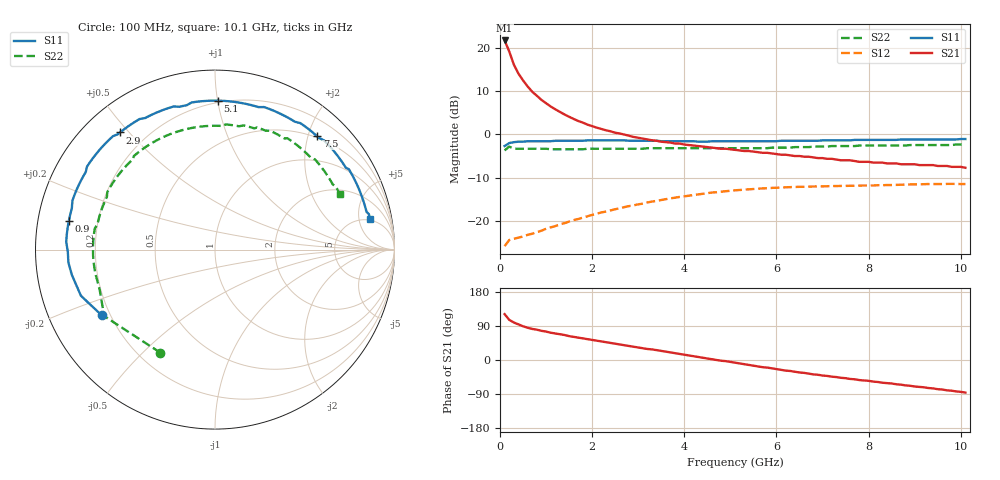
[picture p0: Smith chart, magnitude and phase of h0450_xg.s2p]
!HBFP-0450
!S and NOISE PARAMETERS at Vce=0.5V  Ic=35mA.  LAST UPDATED  09-04-98
# GHZ S MA R  50
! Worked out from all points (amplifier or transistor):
!   101 points, 100 MHz to 10.1 GHz, reference 50 ohm
!   highest |S21| = 21.6 dB at 100 MHz (marker M1)
!   |S21| within 3 dB of that: start of sweep to 215.6 MHz
!   unconditionally stable (mu >= 1): 1.433 GHz to end of sweep
!   at 1.7 GHz: K = 1.06, MAG = 9.9 dB, |S12| = -19.6 dB
!   at 5.1 GHz: K = 1.15, MAG = 2.3 dB, |S12| = -13.0 dB
!   at 10.1 GHz: K = 1.12, MAG = -0.3 dB, |S12| = -11.5 dB
!   lowest NFmin = 1.72 dB at 1.8 GHz
!   S11 on the Smith chart (normalised r, x): 100 MHz: 0.17, -0.26; 900 MHz: 0.09, +0.10; 2.9 GHz: 0.11, +0.47; 5.1 GHz: 0.19, +1.00; 7.5 GHz: 0.47, +2.16; 10.1 GHz: 4.83, +7.19
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0.1  0.73 -150.0  12.09 121.0  0.051 30.0  0.65 -118.0
0.2  0.79 -161.0  9.04 106.0  0.06 22.0  0.72 -149.0
0.3  0.81 -170.0  6.37 99.0  0.062 20.0  0.68 -161.0
0.4  0.82 -175.0  5.01 94.0  0.064 20.0  0.68 -169.0
0.5  0.82 -179.0  4.18 89.0  0.066 21.0  0.68 -174.0
0.6  0.83 177.0  3.56 85.0  0.069 21.0  0.68 -177.0
0.7  0.83 174.0  3.09 82.0  0.071 23.0  0.68 179.0
0.9  0.83 169.0  2.49 77.0  0.077 25.0  0.68 173.0
1.1  0.83 164.0  2.09 72.0  0.084 27.0  0.67 168.0
1.3  0.84 159.0  1.81 68.0  0.091 28.0  0.67 163.0
1.5  0.84 155.0  1.59 63.0  0.098 28.0  0.67 159.0
1.8  0.84 149.0  1.36 57.0  0.109 28.0  0.67 154.0
2.3  0.85 139.0  1.11 47.0  0.128 26.0  0.68 145.0
2.9  0.84 129.0  0.93 35.0  0.151 21.0  0.68 136.0
3.5  0.83 118.0  0.82 24.0  0.174 14.0  0.69 126.0
4.4  0.82 102.0  0.72 6.0  0.205 2.0  0.69 111.0
5.1  0.83 89.0  0.66 -7.0  0.225 -8.0  0.69 99.0
5.7  0.83 78.0  0.61 -19.0  0.237 -17.0  0.69 88.0
6.8  0.84 59.0  0.54 -38.0  0.249 -33.0  0.72 71.0
7.5  0.85 48.0  0.5 -48.0  0.253 -43.0  0.73 61.0
8.5  0.86 34.0  0.46 -62.0  0.259 -55.0  0.74 48.0
10.1  0.88 11.0  0.41 -86.0  0.266 -78.0  0.76 24.0
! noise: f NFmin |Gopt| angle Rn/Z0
1.8  1.72  0.66  -157  0.07
2  1.82  0.64  -153  0.09
2.5  1.81  0.67  -144  0.15
3.5  2.07  0.69  -126  0.32
4  2.15  0.7  -116  0.48
5  2.33  0.71  -97  0.79
5.5  2.43  0.73  -87  1.06
7  2.68  0.75  -59  1.97
8  2.82  0.77  -44  2.4
10  3.19  0.8  -14  3.67
